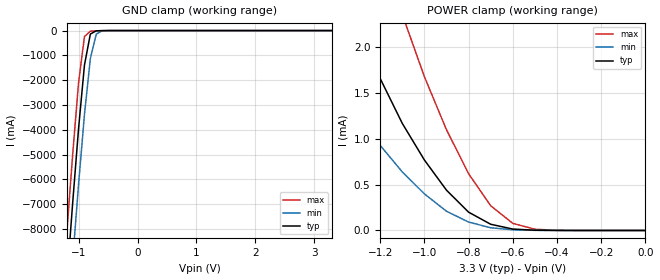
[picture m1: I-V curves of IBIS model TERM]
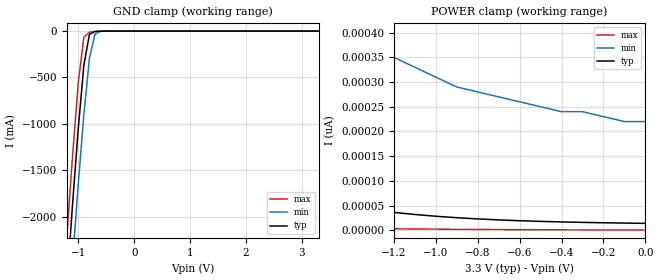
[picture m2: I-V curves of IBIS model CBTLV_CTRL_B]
| I/O Buffer Information Specification (IBIS) Version 3.2 (August 20, 1999)
| IBIS is a standard for electronic behavioral specifications of integrated
| circuit input/output analog characteristics.
[IBIS Ver]   3.2
[File Name]   cbtlv3384.ibs
[File Rev]   1.1
[Date]   Tuesday, October 16 2001
[Source]   Integrated Device Technology, Inc.
[Notes]   1.Temperatures: typ=25C, min=-40C, max=100C
[Disclaimer] Integrated Device Technology, Inc. ("IDT") hereby grants the
   user of this IBIS model a non-exclusive, nontransferable
   license to use this IBIS model under the following terms. The
   user is granted this license only to use the IBIS model and is
   not granted rights to sell, copy (except as needed to run the
   IBIS model), rent, lease or sub-license the IBIS model in
   whole or in part, or in modified form to anyone. The User may
   modify the IBIS model to suit its specific applications, but
   rights to derivative works and such modifications shall belong
   to IDT.
   This IBIS model is provided on an AS IS" basis and IDT
   makes absolutely no warranty with respect to the information
   contained herein. IDT DISCLAIMS AND CUSTOMER WAIVES ALL
   WARRANTIES, EXPRESS AND IMPLIED, INCLUDING WARRANTIES OF
   MERCHANTABILITY AND FITNESS FOR A PARTICULAR PURPOSE. THE
   ENTIRE RISK AS TO QUALITY AND PERFORMANCE IS WITH THE USER
   ACCORDINGLY, IN NO EVENT SHALL IDT BE LIABLE FOR ANY DIRECT OR
   INDIRECT DAMAGES, WHETHER IN CONTRACT OR TORT,  INCLUDING
   ANY LOST PROFITS OR OTHER INCIDENTAL, CONSEQUENTIAL, EXEMPLARY,
   OR PUNITIVE DAMAGES ARISING OUT OF THE USE OR APPLICATION OF
   THE IBIS model.
   Further, IDT reserves the right to make changes without notice
   to any product herein to improve reliability, function, or
   design. IDT does not convey any license under patent rights or
   any other intellectual property rights, including those of
   third parties. IDT is not obligated to provide maintenance or
   support for the licensed IBIS model.
[Copyright]   Copyright 1997, Integrated Device Technology, Inc. all rights
   reserved
|   Component IDT74CBTLV3384
[Component]   IDT74CBTLV3384
[Manufacturer]   Integrated Device Technology
[Package]
|Following package parameters are for SSOP 24 lead package
| variable   typ   min   max
R_pkg   4.00m   2.00m   5.00m
L_pkg   5.01nH   4.65nH   6.05nH
C_pkg   0.045pF   0.035pF   0.067pF
[Pin]  signal_name   model_name   R_pin   L_pin   C_pin
1   _1OE_   CBTLV_CTRL_B
2   1B1   TERM
3   1A1   TERM
4   1A2   TERM
5   1B2   TERM
6   1B3   TERM
7   1A3   TERM
8   1A4   TERM
9   1B4   TERM
10   1B5   TERM
11   1A5   TERM
12   GND   GND
13   _2OE_   CBTLV_CTRL_B
14   2A1   TERM
15   2B1   TERM
16   2B2   TERM
17   2A2   TERM
18   2A3   TERM
19   2B3   TERM
20   2B4   TERM
21   2A4   TERM
22   2A5   TERM
23   2B5   TERM
24   VCC   POWER
| oeb  oeb   dummy_model
[Series Switch Groups]
|Function Group States
On A /
On B /
On A B /
Off A B /
[Series Pin Mapping]   pin_2   model_name   function_table_group
3   2   CBTLV_SW   A
4   5   CBTLV_SW   A
7   6   CBTLV_SW   A
8   9   CBTLV_SW   A
11   10   CBTLV_SW   A
14   15   CBTLV_SW   B
17   16   CBTLV_SW   B
18   19   CBTLV_SW   B
21   20   CBTLV_SW   B
22   23   CBTLV_SW   B
|   Model CBTLV_SW
[Model]   CBTLV_SW
Model_type   Series_switch
C_comp   0.00pF   0.00pF   0.00pF
[Temperature Range]   25.00   100.00   -40.00
[Voltage Range]   3.30V   3.00V   3.6V
[On]
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[Off]
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| Models and submodels in the file (3): TERM (Terminator), CBTLV_CTRL_B (Input), CBTLV_SW (Series_switch)
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|   Model TERM
[Model]   TERM
Model_type   Terminator
Polarity   Non-Inverting
C_comp   5.00pF   5.00pF   5.00pF
[Temperature Range]   25.00   100.00   -40.00
[Voltage Range]   3.30V   3.00V   3.60V
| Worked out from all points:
|   GND clamp passes 1 mA (typ) near -0.54 V on its own axis
|   POWER clamp passes 1 mA (typ) near -1.06 V on its own axis
[GND_clamp]
| voltage   I(typ)   I(min)   I(max)
-3.3V     -82.19A    -84.14A    -80.6A
-1.2V     -10.13A    -12.44A    -8.17A
-1.1V     -6.95A     -9.26A     -5A
-1V       -3.95A     -6.2A      -2.1A
-900mV    -1.39A     -3.38A     -240mA
-800mV    -140mA     -1.13A     -23mA
-700mV    -10.38mA   -140mA     -11.02mA
-600mV    -2.14mA    -10.9mA    -3.97mA
3.3V      43.59pA    38.63nA    59.54pA
[POWER_clamp]
| voltage   I(typ)   I(min)   I(max)
-3.3V     19.83mA    14.03mA    24.7mA
-1.6V     4.15mA     2.52mA     6.59mA
-1.5V     3.45mA     2.06mA     5.66mA
-1.3V     2.2mA      1.26mA     3.9mA
-1.1V     1.17mA     640uA      2.36mA
-1V       770uA      400uA      1.68mA
-900mV    440uA      210uA      1.1mA
-800mV    200uA      91.79uA    620uA
-700mV    67.88uA    29.64uA    270uA
-600mV    15.52uA    7.26uA     77.81uA
-500mV    2.7uA      1.47uA     13.43uA
0V        43.57pA    640pA      91.39pA
|   Model CBTLV_CTRL_B
[Model]   CBTLV_CTRL_B
Model_type   Input
Vinl =   0.80V
Vinh =   2.00V
C_comp   5.00pF   5.00pF   5.00pF
[Temperature Range]   25.00   100.00   -40.00
[Voltage Range]   3.30V   3.00V   3.60V
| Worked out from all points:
|   GND clamp passes 1 mA (typ) near -0.58 V on its own axis
[GND_clamp]
| voltage   I(typ)   I(min)   I(max)
-3.3V     -22A       -22.54A    -21.56A
-1.2V     -2.71A     -3.33A     -2.18A
-1.1V     -1.85A     -2.47A     -1.33A
-1V       -1.05A     -1.65A     -560mA
-900mV    -370mA     -900mA     -66.52mA
-800mV    -35.18mA   -290mA     -11.47mA
-700mV    -4.02mA    -32.89mA   -5.96mA
-600mV    -1.16mA    -2.31mA    -2.17mA
3.3V      14.11pA    240pA      630fA
[POWER_clamp]
| voltage   I(typ)   I(min)   I(max)
-3.3V     620pA      3.78nA     60.89pA
-3V       430pA      2.65nA     42.48pA
-2.9V     380pA      2.34nA     37.5pA
-2.6V     260pA      1.61nA     25.42pA
-2.3V     170pA      1.1nA      16.85pA
-2V       110pA      760pA      10.91pA
-1.8V     84.03pA    610pA      8.09pA
-1.4V     47.41pA    410pA      4.34pA
-1.2V     36.31pA    350pA      3.19pA
-900mV    25.54pA    290pA      2.02pA
-400mV    16.97pA    240pA      1.06pA
0V        14.1pA     220pA      750fA
